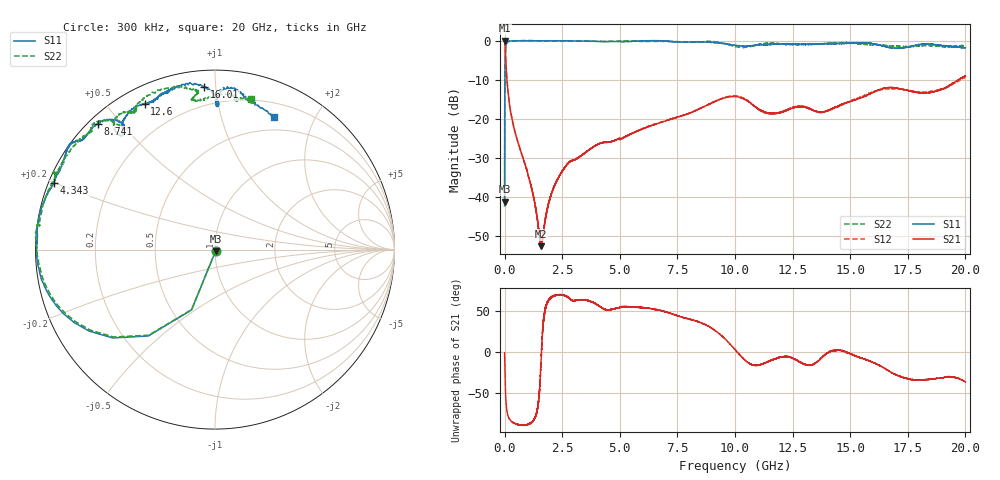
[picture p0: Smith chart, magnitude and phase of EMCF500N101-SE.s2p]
!EMCF500N101
!Johanson Technology Inc.
!www.johansontechnology.com
!Test Board Conditions:
!Substrate Type  RO4350B
!Substrate Thickness  6.6 mil
!Substrate Dk  3.66
!TL Type: GCPW
!TL Trace Width  13 mil
!TL Gap  7.5 mil
!PART MODE SINGLE ENDED (AKA BYPASS)
!DUT TOPOLOGY	SERIES-SHUNT
# MHz S  dB  R 50
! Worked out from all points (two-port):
!   20001 points, 300 kHz to 20 GHz, reference 50 ohm
!   highest |S21| = 0.01 dB at 300 kHz (marker M1); lowest = -52.7 dB at 1.589 GHz (marker M2)
!   |S21| within 3 dB of the highest: start of sweep to 33.93 MHz
!   lowest |S11| = -41.3 dB at 300 kHz (marker M3), VSWR 1.02, Z = 50.4 - j0.783 ohm
!   |S11| at or under -10 dB: start of sweep to 11.46 MHz
!   |S22| runs from -42.5 to 0.0 dB; largest |S21 - S12| = 0.017
!   S11 on the Smith chart (normalised r, x): 300 kHz: 1.01, -0.02; 4.343 GHz: 0.02, +0.20; 8.741 GHz: 0.03, +0.43; 12.6 GHz: 0.07, +0.63; 16.01 GHz: 0.09, +0.93; 20 GHz: 0.34, +1.48
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0.3  -41.28 -64.3  0.01 -0.8  0.03 -0.7  -42.53 -64.1
101.298  -0.48 -162.1  -9.96 -71.6  -9.92 -71.6  -0.56 -162.1
134.298  -0.29 -166.7  -12.26 -76.1  -12.20 -76.1  -0.38 -166.7
359.295  -0.05 -176.8  -21.17 -85.5  -21.16 -85.6  -0.10 -177.7
1165.283  -0.06 177.1  -37.58 -85.6  -37.63 -84.9  -0.00 172.3
1589.276  -0.04 174.2  -52.66 -6.3  -52.10 -6.9  -0.07 171.9
1927.271  -0.02 171.4  -41.26 63.6  -41.27 64.0  -0.11 172.2
2236.266  -0.03 168.9  -36.24 69.5  -36.19 68.5  -0.10 172.0
2752.259  -0.07 165.5  -31.45 66.6  -31.42 66.2  -0.09 169.3
3334.25  -0.10 163.1  -29.38 63.4  -29.42 63.5  -0.09 163.9
4343.235  -0.26 157.6  -26.08 51.9  -26.06 51.9  -0.21 156.2
6667.2  -0.03 143.6  -21.18 51.2  -21.14 50.9  -0.17 149.8
8741.169  -0.38 133.0  -16.66 33.0  -16.71 32.8  -0.25 135.0
10000.15  -1.21 126.2  -14.31 3.1  -14.12 3.4  -1.50 127.5
11392.13  -1.00 124.2  -18.48 -12.1  -18.62 -11.3  -0.70 126.4
12599.11  -0.90 115.7  -17.07 -8.7  -16.97 -8.8  -1.06 120.3
13334.1  -0.94 111.7  -17.72 -15.6  -17.63 -16.0  -0.97 119.4
14302.08  -0.74 107.5  -17.18 1.8  -17.27 1.7  -0.66 115.8
16009.06  -0.85 93.9  -13.21 -12.9  -13.15 -14.4  -1.09 96.0
16667.05  -1.77 88.8  -12.02 -22.8  -12.35 -23.2  -1.33 97.8
18461.02  -0.86 83.1  -13.33 -33.0  -13.06 -33.9  -1.27 83.4
20000  -1.82 66.2  -9.07 -36.3  -9.31 -34.5  -1.30 76.6
